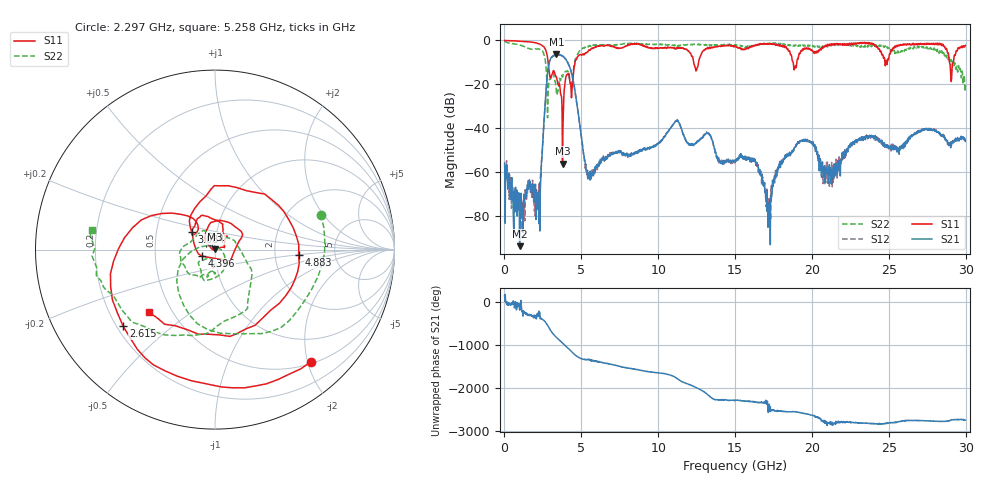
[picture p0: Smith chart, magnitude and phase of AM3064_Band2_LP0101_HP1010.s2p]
# Hz S DB R 50.0
!freq dBS11 angS11 dBS21 angS21 dBS12 angS12 dBS22 angS22
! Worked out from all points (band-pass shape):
!   1600 points, 10 MHz to 29.98 GHz, reference 50 ohm
!   highest |S21| = -6.40 dB at 3.384 GHz (marker M1); lowest = -93.8 dB at 984.7 MHz (marker M2)
!   |S21| within 3 dB of the highest: 2.943 GHz to 4.058 GHz (1.114 GHz wide, 31.8 % of centre)
!   lowest |S11| = -56.1 dB at 3.777 GHz (marker M3), VSWR 1.00, Z = 49.9 + j0.135 ohm
!   |S11| at or under -10 dB: 2.84 GHz to 4.591 GHz (1.751 GHz wide, 47.1 % of centre); 12.3 GHz to 12.62 GHz (319.4 MHz wide, 2.56 % of centre); 28.94 GHz to 29.2 GHz (255.5 MHz wide, 0.879 % of centre)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
!   |S22| runs from -35.3 to -0.3 dB; largest |S21 - S12| = 0.015
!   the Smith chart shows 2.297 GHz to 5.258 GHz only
!   S11 on the Smith chart (normalised r, x): 2.297 GHz: 0.53, -2.06; 2.615 GHz: 0.23, -0.35; 3.084 GHz: 0.76, +0.16; 4.396 GHz: 0.87, -0.06; 4.883 GHz: 2.73, -0.20; 5.258 GHz: 0.37, -0.35
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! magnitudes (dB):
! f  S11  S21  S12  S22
! 10 MHz  0.0  -55.9  -57.9  -0.3
! 984.7 MHz  -0.4  -93.8  -80.4  -2.1
! 2.297 GHz  -1.7  -86.9  -64.9  -4.2
! 2.615 GHz  -3.5  -32.2  -32.2  -7.5
! 3.084 GHz  -15.7  -7.6  -7.5  -15.9
! 3.384 GHz  -16.7  -6.4  -6.4  -24.0
! 3.777 GHz  -56.1  -7.2  -7.1  -16.7
! 4.396 GHz  -22.0  -15.9  -15.9  -18.5
! 4.883 GHz  -6.6  -37.8  -37.7  -4.8
! 5.015 GHz  -6.8  -44.7  -44.4  -4.2
! 5.258 GHz  -5.9  -56.1  -58.3  -3.2
! 10 GHz  -3.5  -46.7  -46.9  -1.9
! 11.24 GHz  -3.7  -36.8  -36.6  -2.6
! 15 GHz  -2.7  -55.3  -55.3  -2.0
! 16.35 GHz  -2.2  -56.6  -57.0  -2.4
! 17.2 GHz  -1.5  -74.5  -77.8  -1.7
! 18.04 GHz  -2.4  -55.7  -55.5  -2.0
! 19.99 GHz  -4.4  -46.9  -46.8  -2.3
! 21.27 GHz  -1.5  -65.5  -63.0  -2.2
! 23.18 GHz  -0.9  -44.6  -44.9  -2.7
! 25 GHz  -8.3  -48.7  -48.9  -3.2
! 29.98 GHz  -2.3  -46.1  -45.9  -20.3
